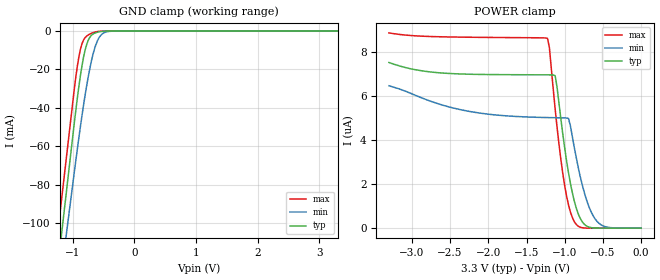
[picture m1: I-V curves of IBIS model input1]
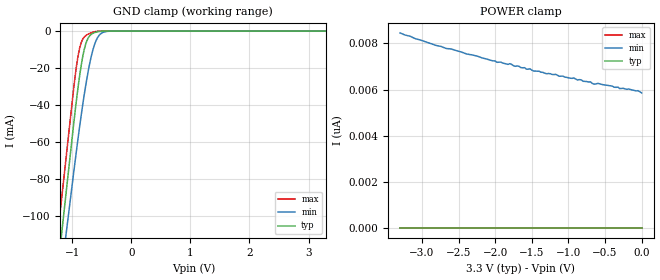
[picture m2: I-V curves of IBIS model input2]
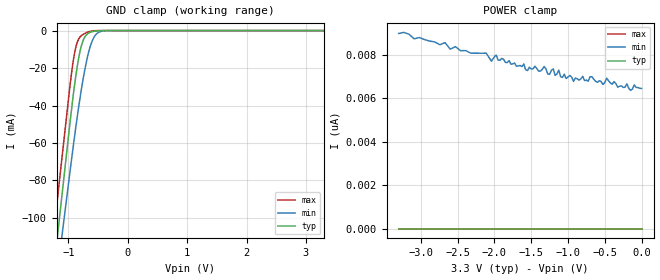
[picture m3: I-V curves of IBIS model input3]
|   Microchip Technology Inc.
|   93LC86C - 16 Kbit Microwire serial EEPROM
|   (Vcc = +2.5V to +5.5V)
|   150K Process
|   Copyright (C) 2018 Microchip Technology Inc.
[IBIS ver]   3.2
[File name]   93lc86c-e_st-3_3v.ibs
[File Rev]   1.0
[Date]   May 18, 2018
[Source]   Waveforms generated by SPICE simulation at Microchip.
   All other data taken from lab measurements at Microchip.
[Notes]   This IBIS model is for the Microchip 93LC86C device, a
   16 Kbit Microwire bus serial EEPROM manufactured on
   Microchip's 150K process, for automotive temp in
   a 4.4 mm, 8-lead TSSOP package operating at 3.3V.
[Disclaimer] Unauthorized reproduction and/or distribution is
   strictly restricted. All rights reserved.
   This information is provided to you for your convenience
   and use with Microchip products only. Microchip
   disclaims all liability arising from this information
   and its use.
   THIS INFORMATION IS PROVIDED "AS IS." MICROCHIP MAKES NO
   REPRESENTATION OR WARRANTIES OF ANY KIND WHETHER EXPRESS
   OR IMPLIED, WRITTEN OR ORAL, STATUTORY OR OTHERWISE,
   RELATED TO THE INFORMATION PROVIDED TO YOU, INCLUDING
   BUT NOT LIMITED TO ITS CONDITION, QUALITY, PERFORMANCE,
   MERCHANTABILITY, NON-INFRINGEMENT, OR FITNESS FOR
   PURPOSE. MICROCHIP IS NOT LIABLE, UNDER ANY
   CIRCUMSTANCES, FOR SPECIAL, INCIDENTAL OR CONSEQUENTIAL
   DAMAGES, FOR ANY REASON WHATSOEVER.
   It is your responsibility to ensure that your
   application meets with your specifications.
|   Component 93LC86C-E/ST
[Component]   93LC86C-E/ST
[Manufacturer]   Microchip Technology Inc.
[Package]
| variable   typ   min   max
R_pkg   99.09m   85.92m   112.26m
L_pkg   2.16nH   1.55nH   2.76nH
C_pkg   0.49pF   0.43pF   0.55pF
[Pin]  signal_name   model_name
1   CS   input1
2   CLK   input2
3   DI   input3
4   DO   driver
5   VSS   GND
6   ORG   input4
7   PE   input5
8   VCC   POWER
| Models and submodels in the file (6): input1 (Input), input2 (Input), input3 (Input), driver (3-state), input4 (Input), input5 (Input)
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|   Model input1
[Model]   input1
Model_type   Input
Vinl = 0.8
Vinh = 2.0
C_comp   5.00pF   5.00pF   5.00pF
[Temperature Range]   25.00   125.00   -40.00
[Voltage Range]   3.30V   2.50V   5.50V
[Pullup Reference]   3.30V   3.30V   3.30V
[POWER Clamp Reference]   3.30V   3.30V   3.30V
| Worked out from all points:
|   GND clamp passes 1 mA (typ) near -0.64 V on its own axis
[GND_clamp]
| voltage   I(typ)   I(min)   I(max)
-3.3V     -698.8mA   -657.5mA   -676.5mA
-1.26V    -127.6mA   -145mA     -109.4mA
-1.175V   -103.8mA   -123.7mA   -85.74mA
-1.09V    -80mA      -102.3mA   -62.11mA
-975mV    -47.8mA    -73.44mA   -30.14mA
-900mV    -28.63mA   -55.3mA    -13.23mA
-850mV    -17.97mA   -43.91mA   -6.539mA
-800mV    -9.884mA   -33.36mA   -3.4mA
-725mV    -3.301mA   -19.74mA   -1.553mA
-600mV    -588.4uA   -5.069mA   -233.5uA
-425mV    -8.051uA   -236.5uA   -371.5nA
3.3V      10pA       3.662nA    10pA
[POWER_clamp]
| voltage   I(typ)   I(min)   I(max)
-3.3V     7.505uA    6.448uA    8.844uA
-2.32V    6.979uA    5.336uA    8.65uA
-1.225V   6.944uA    5.009uA    8.594uA
-1.2V     6.943uA    5.007uA    8.166uA
-1.125V   6.906uA    5.002uA    5.394uA
-1V       3.626uA    4.994uA    1.92uA
-950mV    2.499uA    4.966uA    1.046uA
-875mV    1.23uA     3.662uA    296.9nA
-800mV    462.5nA    2.382uA    46.96nA
-725mV    120.2nA    1.394uA    4.568nA
-575mV    3.035nA    298.9nA    10pA
0V        10pA       5.241nA    10pA
|   Model input2
[Model]   input2
Model_type   Input
Vinl = 0.8
Vinh = 2.0
C_comp   5.00pF   5.00pF   5.00pF
[Temperature Range]   25.00   125.00   -40.00
[Voltage Range]   3.30V   2.50V   5.50V
[Pullup Reference]   3.30V   3.30V   3.30V
[POWER Clamp Reference]   3.30V   3.30V   3.30V
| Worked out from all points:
|   GND clamp passes 1 mA (typ) near -0.64 V on its own axis
[GND_clamp]
| voltage   I(typ)   I(min)   I(max)
-3.3V     -725mA     -676.9mA   -708.6mA
-1.26V    -132.6mA   -149.8mA   -113.7mA
-1.175V   -107.9mA   -127.8mA   -88.95mA
-1.09V    -83.2mA    -105.8mA   -64.16mA
-975mV    -49.8mA    -76.11mA   -30.63mA
-900mV    -29.88mA   -57.47mA   -13.1mA
-850mV    -18.78mA   -45.75mA   -6.36mA
-800mV    -10.29mA   -34.87mA   -3.324mA
-725mV    -3.382mA   -20.77mA   -1.528mA
-600mV    -592.5uA   -5.376mA   -221.7uA
-425mV    -8.179uA   -241.6uA   -312.7nA
3.3V      10pA       4.121nA    10pA
[POWER_clamp]
| voltage   I(typ)   I(min)   I(max)
-3.3V     10pA       8.448nA    10pA
-2.81V    10pA       7.908nA    10pA
-1.975V   10pA       7.176nA    10pA
-1.8V     10pA       7.118nA    10pA
-1.3V     10pA       6.683nA    10pA
-925mV    10pA       6.499nA    10pA
-700mV    10pA       6.332nA    10pA
-650mV    10pA       6.235nA    10pA
-600mV    10pA       6.267nA    10pA
-300mV    10pA       6.04nA     10pA
-50mV     10pA       5.952nA    10pA
0V        10pA       5.852nA    10pA
|   Model input3
[Model]   input3
Model_type   Input
Vinl = 0.8
Vinh = 2.0
C_comp   5.00pF   5.00pF   5.00pF
[Temperature Range]   25.00   125.00   -40.00
[Voltage Range]   3.30V   2.50V   5.50V
[Pullup Reference]   3.30V   3.30V   3.30V
[POWER Clamp Reference]   3.30V   3.30V   3.30V
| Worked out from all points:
|   GND clamp passes 1 mA (typ) near -0.64 V on its own axis
[GND_clamp]
| voltage   I(typ)   I(min)   I(max)
-3.3V     -716.5mA   -665.4mA   -695.6mA
-1.26V    -131.4mA   -148mA     -111.4mA
-1.175V   -107mA     -126.5mA   -87.05mA
-1.09V    -82.64mA   -104.9mA   -62.71mA
-975mV    -49.66mA   -75.73mA   -29.77mA
-900mV    -29.95mA   -57.38mA   -12.62mA
-850mV    -18.91mA   -45.83mA   -6.134mA
-800mV    -10.43mA   -35.08mA   -3.255mA
-725mV    -3.441mA   -21.09mA   -1.508mA
-600mV    -602uA     -5.595mA   -215.6uA
-425mV    -8.622uA   -258.3uA   -289.3nA
3.3V      10pA       4.543nA    10pA
[POWER_clamp]
| voltage   I(typ)   I(min)   I(max)
-3.3V     10pA       8.969nA    10pA
-2.11V    10pA       8.064nA    10pA
-2.04V    10pA       7.696nA    10pA
-1.975V   10pA       7.98nA     10pA
-1.55V    10pA       7.269nA    10pA
-1.125V   10pA       7.289nA    10pA
-925mV    10pA       6.771nA    10pA
-675mV    10pA       6.982nA    10pA
-525mV    10pA       6.631nA    10pA
-475mV    10pA       6.921nA    10pA
-325mV    10pA       6.506nA    10pA
0V        10pA       6.447nA    10pA
